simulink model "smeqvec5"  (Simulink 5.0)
settings: Solver=ode23t  StartTime=0.0  StopTime=40  MaxStep=0.05  RelTol=1e-3  AbsTol=1e-3
InitFcn:
  | smvecdef5
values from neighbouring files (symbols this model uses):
  Bm = 0.10    (= 0.1)    [IMabc2.m]    (also in imabcparam.m = 0.01; IMabcrun0.m = 0.01; IMabcrun1.m = 0.001; IMcur0.m = 1e-06)
  H = 0.60    (= 0.6)    [IMabc2.m]    (also in IMcur0.m = 0.3; imdef0vec.m = 0.3; imdef1vec.m = 0.3; imdef2vec.m = 0.3)
  n0 = 0.98    [imdef0vec.m]    (also in imdef1vec.m = 0.978; imdef2vec.m; imdefrotflux.m; imdefSIvec1.m = 0.95)
  Ra = .95    (= 0.95)    [altwdgs.m]    (also in Ccurverun.m = 0.018)
  wo = 2*pi*freq0    [calc0.m]    (also in IMabc2.m = 376.991118431; imabcparam.m = 376.991118431; IMabcrun0.m = 376.991118431; IMabcrun1.m = 376.991118431)
undefined symbols (not defined in the file or in its folder): delta0, fa0, fk0, L_1, phif0, Rf, Rkd, Rkq, vf0
libraries: simulink x1

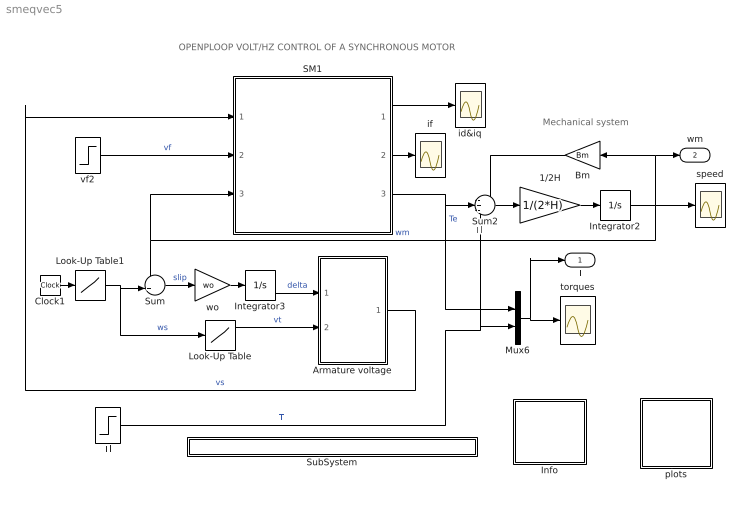
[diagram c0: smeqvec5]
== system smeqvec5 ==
  note: Tl
  note: OPENPLOOP VOLT/HZ CONTROL OF A SYNCHRONOUS MOTOR
  note: Mechanical system
  1/2H : Gain  Gain=1/(2*H)
  Armature voltage : Subsystem
  Bm : Gain  Orientation=left  Gain=Bm
  Clock1 : Clock
  Info : Subsystem
  Integrator2 : Integrator  InitialCondition=n0
  Integrator3 : Integrator  InitialCondition=delta0
  Look-Up Table : Lookup  InputValues=[-1 0 1]  OutputValues=[1 0.04 1]
  Look-Up Table1 : Lookup  InputValues="[0  10 25 30 40]"  OutputValues="[0  1 1 0.8 0.8]"
  Mux6 : Mux  Inputs=2
  SM1 : Subsystem
  SubSystem : Subsystem
  Sum : Sum  Inputs=-+|
  Sum2 : Sum  Inputs=-+-
  Tl : Step  Time=17.5  After=0.6  SampleTime=0
  id&iq : Scope
  if : Scope
  plots : Subsystem
  speed : Scope
  torques : Scope
  vf2 : Step  Before=vf0  After=vf0  SampleTime=0
  wo : Gain  Gain=wo
  T : Outport
  wm : Outport  Port=2
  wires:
  vf2/1 -> SM1/2(vf)  "vf"
  1/2H/1 -> Integrator2/1
  Bm/1 -> Sum2/1
  SM1/3(Te) -> Mux6/1, Sum2/2  "Te"
  Sum/1 -> wo/1  "slip"
  wo/1 -> Integrator3/1
  Integrator3/1 -> Armature voltage/1(delta)  "delta"
  Integrator2/1 -> Sum/1, SM1/3(wm), speed/1, Bm/1, wm/1  "wm"
  Tl/1 -> Mux6/2, Sum2/3  "Tl"
  Look-Up Table/1 -> Armature voltage/2(Vt)  "vt"
  Look-Up Table1/1 -> Sum/2, Look-Up Table/1  "ws"
  Armature voltage/1(vs) -> SM1/1(vs)  "vs"
  SM1/2(if) -> if/1
  Mux6/1 -> torques/1, T/1
  SM1/1(ia) -> id&iq/1
  Sum2/1 -> 1/2H/1
  Clock1/1 -> Look-Up Table1/1

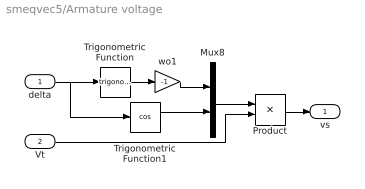
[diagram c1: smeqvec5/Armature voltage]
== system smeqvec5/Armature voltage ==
  delta : Inport
  Vt : Inport  Port=2
  Mux8 : Mux  Inputs=2
  Product : Product
  Trigonometric Function : Trigonometry
  Trigonometric Function1 : Trigonometry  Operator=cos
  wo1 : Gain  Gain=-1
  vs : Outport
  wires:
  delta/1 -> Trigonometric Function/1, Trigonometric Function1/1
  Trigonometric Function/1 -> wo1/1
  Mux8/1 -> Product/1
  wo1/1 -> Mux8/1
  Trigonometric Function1/1 -> Mux8/2
  Product/1 -> vs/1
  Vt/1 -> Product/2

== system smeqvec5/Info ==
  note: Open-loop Volt/Hz control of a synchronous motor

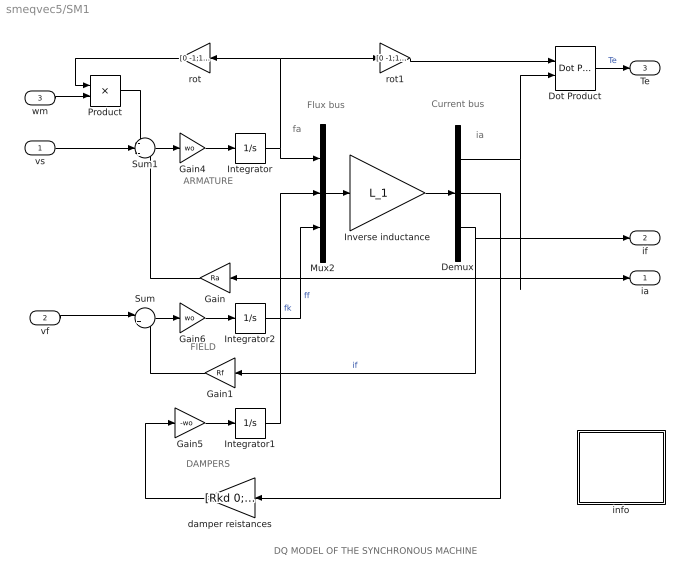
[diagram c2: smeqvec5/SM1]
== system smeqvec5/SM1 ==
  note: DAMPERS
  note: ARMATURE
  note: fa
  note: ia
  note: FIELD
  note: DQ MODEL OF THE SYNCHRONOUS MACHINE
  note: Flux bus
  note: Current bus
  vs : Inport
  vf : Inport  Port=2
  wm : Inport  Port=3
  Demux : Demux  Outputs=3
  Dot Product : simulink/Math Operations/Dot Product
  Gain : Gain  Orientation=left  Gain=Ra
  Gain1 : Gain  Orientation=left  Gain=Rf
  Gain4 : Gain  Gain=wo
  Gain5 : Gain  Gain=-wo
  Gain6 : Gain  Gain=wo
  Integrator : Integrator  InitialCondition=fa0
  Integrator1 : Integrator  InitialCondition=fk0
  Integrator2 : Integrator  InitialCondition=phif0
  Inverse inductance : Gain  Gain=L_1  Multiplication=Matrix(K*u)
  Mux2 : Mux  Inputs=3
  Product : Product
  Sum : Sum  Inputs=|+-
  Sum1 : Sum  Inputs=-+-
  damper reistances : Gain  Orientation=left  Gain=[Rkd 0;0 Rkq]  Multiplication=Matrix(K*u)
  info : Subsystem
  rot : Gain  Orientation=left  Gain=[0 -1;1 0]  Multiplication=Matrix(K*u)
  rot1 : Gain  Gain=[0 -1;1 0]  Multiplication=Matrix(K*u)
  ia : Outport
  if : Outport  Port=2
  Te : Outport  Port=3
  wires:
  Product/1 -> Sum1/1
  rot/1 -> Product/1
  wm/1 -> Product/2
  Gain5/1 -> Integrator1/1
  damper reistances/1 -> Gain5/1
  Integrator/1 -> Mux2/1, rot/1, rot1/1
  Sum1/1 -> Gain4/1
  Gain4/1 -> Integrator/1
  vs/1 -> Sum1/2
  Gain/1 -> Sum1/3
  Gain6/1 -> Integrator2/1
  Sum/1 -> Gain6/1
  vf/1 -> Sum/1
  Gain1/1 -> Sum/2
  rot1/1 -> Dot Product/1
  Demux/1 -> Gain/1, ia/1, Dot Product/2
  Mux2/1 -> Inverse inductance/1
  Inverse inductance/1 -> Demux/1
  Integrator1/1 -> Mux2/2  "fk"
  Integrator2/1 -> Mux2/3  "ff"
  Demux/2 -> damper reistances/1
  Demux/3 -> if/1, Gain1/1  "if"
  Dot Product/1 -> Te/1  "Te"

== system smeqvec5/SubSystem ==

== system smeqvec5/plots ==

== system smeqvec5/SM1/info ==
  note: This demonstration illustrates the dynamics of a synchronous generator, initially at no load, following a three-phase short circuit at the terminals.
  note: Synchronous machine transients under shortcircuit
